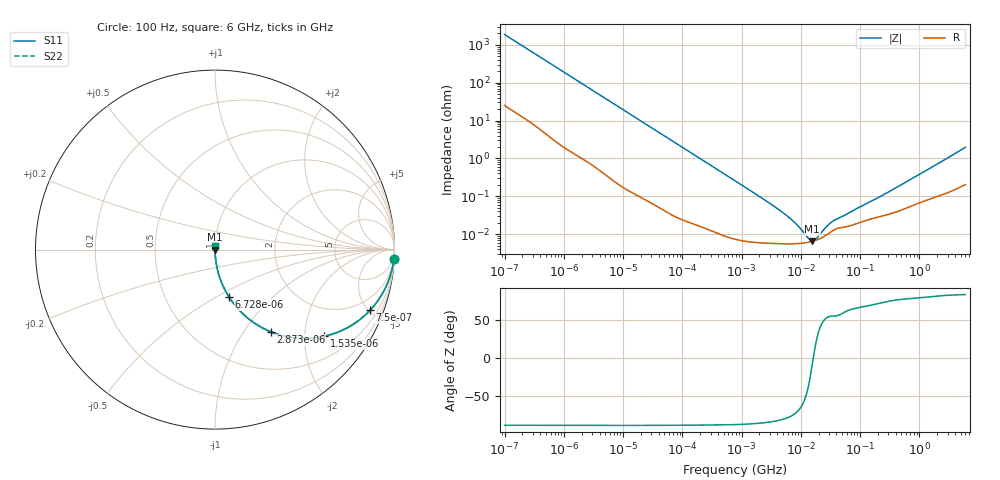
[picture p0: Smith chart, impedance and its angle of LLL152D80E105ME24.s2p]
!Murata Part Number: LLL152D80E105ME24
!These Parameters are Measured in Series Mode Connection
!Data Generated on Jan 08, 2026
!  o--ll--o
!Port1  Port2
!  o------o
!Operation Temp=25[degC], DC Bias Voltage=0[V]
!Freq. Start=100[Hz] Stop=6[GHz] 401[Steps]
# Hz S RI R 50
!Freq.(Hz) S11(Real) S11(Imag) S21(Real) S21(Imag) S12(Real) S12(Imag) S22(Real) S22(Imag)
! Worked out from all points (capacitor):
!   401 points, 100 Hz to 6 GHz, reference 50 ohm
!   read as one part in series: C = 845 nF near 109 Hz
!   lowest |Z| = 6.53 mohm at 15.56 MHz (marker M1)
!   series resonance near 16.24 MHz, so ESL is about 110 pH
!   S11 on the Smith chart (normalised r, x): 100 Hz: 2, -38; 750 Hz: 1.05, -5.09; 1.535 kHz: 1.03, -2.50; 2.873 kHz: 1.01, -1.34; 6.728 kHz: 1.01, -0.58; 6 GHz: 1.00, +0.04
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100  0.9965 -0.053  0.00353 0.053  0.00353 0.053  0.9965 -0.053
293  0.9749 -0.1503  0.0251 0.1503  0.0251 0.1503  0.9749 -0.1503
501  0.9328 -0.2447  0.0672 0.2447  0.0672 0.2447  0.9328 -0.2447
750  0.8637 -0.3379  0.1363 0.3379  0.1363 0.3379  0.8637 -0.3379
1073  0.7584 -0.423  0.2416 0.423  0.2416 0.423  0.7584 -0.423
1535  0.6081 -0.483  0.3919 0.483  0.3919 0.483  0.6081 -0.483
2008  0.4778 -0.4943  0.5222 0.4943  0.5222 0.4943  0.4778 -0.4943
2873  0.3117 -0.458  0.6883 0.458  0.6883 0.458  0.3117 -0.458
4299  0.1703 -0.371  0.8297 0.371  0.8297 0.371  0.1703 -0.371
6728  0.0785 -0.2645  0.9215 0.2645  0.9215 0.2645  0.0785 -0.2645
15062  0.0175 -0.1266  0.9825 0.1266  0.9825 0.1266  0.0175 -0.1266
40335  0.00284 -0.0483  0.9972 0.0483  0.9972 0.0483  0.00284 -0.0483
774597  7.98e-05 -0.00257  0.9999 0.00257  0.9999 0.00257  7.98e-05 -0.00257
4856642  5.55e-05 -0.000377  0.9999 0.000377  0.9999 0.000377  5.55e-05 -0.000377
7599586  5.55e-05 -0.000207  0.9999 0.000207  0.9999 0.000207  5.55e-05 -0.000207
1.189169e7  5.9e-05 -7.83e-05  0.9999 7.83e-05  0.9999 7.83e-05  5.9e-05 -7.83e-05
1.555665e7  6.44e-05 -1.05e-05  0.9999 1.05e-05  0.9999 1.05e-05  6.44e-05 -1.05e-05
2.128304e7  7.68e-05 6.66e-05  0.9999 -6.66e-05  0.9999 -6.66e-05  7.68e-05 6.66e-05
2.911731e7  0.000102 0.000143  0.9999 -0.000143  0.9999 -0.000143  0.000102 0.000143
3.64232e7  0.00013 0.00019  0.9999 -0.00019  0.9999 -0.00019  0.00013 0.00019
3.124326e8  0.000339 0.00129  0.9997 -0.00129  0.9997 -0.00129  0.000339 0.00129
6e9  0.0024 0.0195  0.9976 -0.0195  0.9976 -0.0195  0.0024 0.0195
